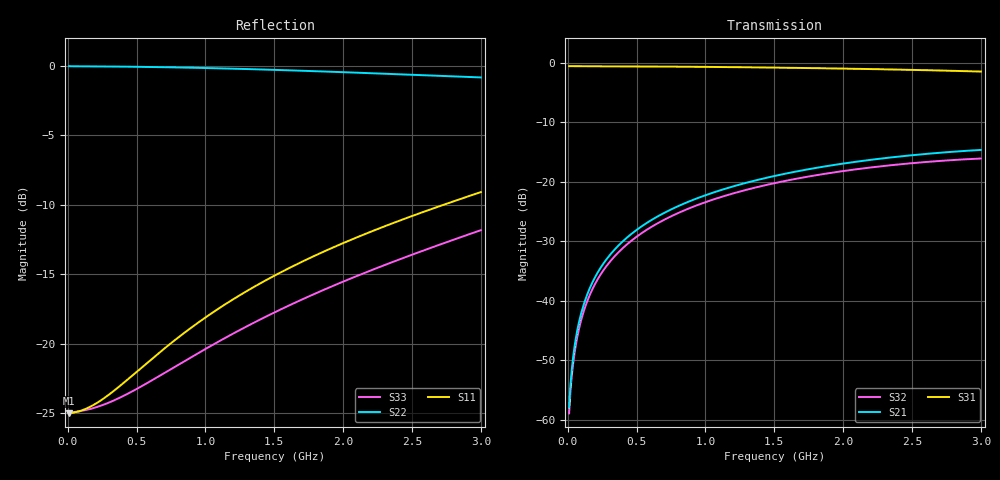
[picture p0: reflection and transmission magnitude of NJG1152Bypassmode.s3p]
! Created Fri Sep 07 18:47:06 2012
# hz S ma R 50
! 3 Port Network Data Port1:RFIN  Port2:RFOUT  Port3:RFOUT2
! freq  magS11  angS11  magS12  angS12  magS13  angS13
!  magS21  angS21
!  magS22  angS22  magS23  angS23
!  magS31  angS31  magS32  angS32
!  magS33  angS33
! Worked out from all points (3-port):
!   300 points, 10 MHz to 3 GHz, reference 50 ohm
!   strongest paths, dB at 10 MHz, 760 MHz, 1.51 GHz, 2.26 GHz, 3 GHz:
!     S31: -0.5, -0.6, -0.8, -1.0, -1.4
!     S21: -57.9, -24.5, -19.0, -16.1, -14.6
!     S32: -58.9, -25.7, -20.2, -17.4, -16.1
!   lowest |S11| = -25.0 dB at 10 MHz (marker M1), VSWR 1.12, Z = 56 - j0.151 ohm
!   |S11| at or under -10 dB: start of sweep to 2.728 GHz
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1e7  0.05629 -1.4  0.001267 63.8  0.9402 -0.2
     0.001274 64.3  0.9966 -0.3  0.001142 64.1
     0.9402 -0.2  0.001135 63.6  0.05663 -1.0
2e7  0.05635 -2.6  0.001963 67.3  0.9401 -0.3
     0.001987 67.8  0.996 -0.5  0.001781 67.7
     0.9401 -0.3  0.00176 67.2  0.05668 -1.9
4e7  0.05657 -5.2  0.003364 74.9  0.94 -0.6
     0.003423 75.3  0.9957 -1.0  0.003068 75.2
     0.94 -0.6  0.003015 74.8  0.05684 -3.8
1e8  0.05762 -12.9  0.007895 81.3  0.9397 -1.5
     0.008057 81.5  0.9955 -2.4  0.007223 81.4
     0.9397 -1.5  0.007079 81.2  0.05741 -9.6
1.9e8  0.06044 -23.8  0.01485 81.9  0.9392 -2.9
       0.01516 82.1  0.995 -4.5  0.01359 82.0
       0.9392 -2.9  0.01331 81.9  0.05885 -18.0
3.3e8  0.0675 -38.7  0.02567 79.7  0.938 -5.1
       0.02621 79.8  0.9937 -7.7  0.02347 80.0
       0.938 -5.1  0.02299 79.9  0.06246 -30.2
5.2e8  0.08089 -54.7  0.0402 75.6  0.9359 -8.0
       0.04105 75.6  0.9912 -12.2  0.03675 76.1
       0.9359 -8.0  0.03599 76.0  0.06971 -44.8
7.8e8  0.1034 -70.5  0.05969 69.4  0.932 -12.0
       0.06097 69.4  0.9866 -18.2  0.05451 70.2
       0.932 -12.0  0.05337 70.2  0.08284 -61.1
1.51e9  0.1769 -97.9  0.1104 51.2  0.9145 -23.2
        0.1128 51.2  0.9664 -35.1  0.1004 53.1
        0.9145 -23.2  0.09819 53.1  0.1304 -92.4
3e9  0.3514 -133.2  0.1811 12.5  0.8472 -47.1
     0.1859 12.5  0.9079 -69.2  0.1616 16.5
     0.8473 -47.1  0.1574 16.5  0.2564 -132.7
